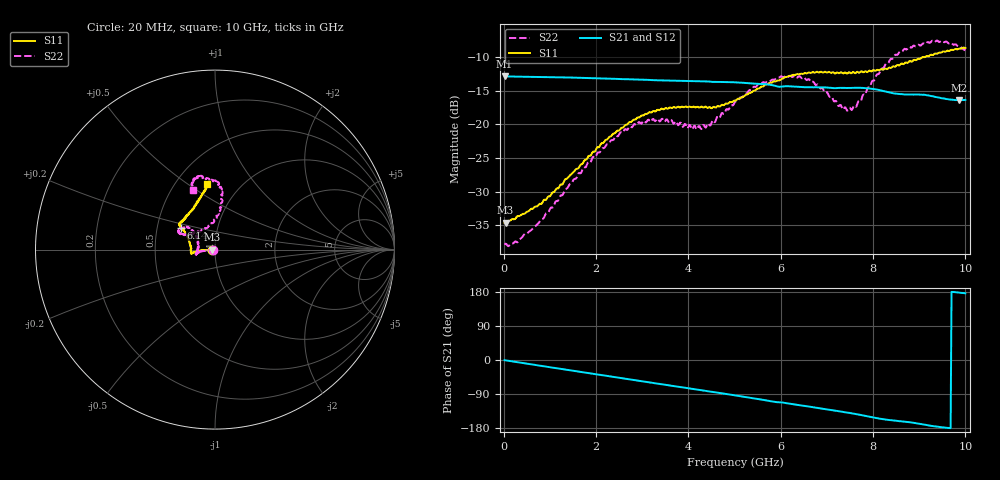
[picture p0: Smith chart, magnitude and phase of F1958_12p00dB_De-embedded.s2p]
! Integrated Device Technology
! Corporate Headquarters
! 6024 Silver Creek Valley Road
! San Jose, CA 95138  USA
! Phone:  1-408-284-8200
! Toll Free:  1-800-223-1366
! Webpage:  http://www.idt.com/
! Timing and RF Division
! 515 Groton Road, Suite 102
! Westford, MA 01886-6024
! Device:  F1958
! Description: 7-bit 0.25 dB Digital Step Attenuator
! Frequency:  0.001 -  6.000 GHz
! Package:  4x4 mm Thin QFN Plastic Package: 24 pin
! Ports:  2 RF, 12 DC
!  Pin  1  = D0
!  Pin  2  = VDD
!  Pin  3  = VMODE
!  Pin  4  = GND
!  Pin  5  = RF1  =  Port 1
!  Pin  6  = GND
!  Pin  7  = GND
!  Pin  8  = GND
!  Pin  9  = GND
!  Pin 10  = GND
!  Pin 11  = GND
!  Pin 12  = GND
!  Pin 13  = GND
!  Pin 14  = RF2  =  Port 2
!  Pin 15  = GND
!  Pin 16  = LE
!  Pin 17  = CLK
!  Pin 18  = DATA
!  Pin 19  = D6
!  Pin 20  = D5
!  Pin 21  = D4
!  Pin 22  = D3
!  Pin 23  = D2
!  Pin 24  = D1
! State:  48
! Atten State:  12.00 dB
! Voltage:  +3.30 Volts
! Current:  0.258 mA
! Data:  The device was measured on a F1958 evaluation board which has
!  individual transmission lines to the RF pins.  Data was collected
!  using a calibrated network analyzer.  The evaluation board was
!  de-embedded using Automatic Fixture Removal (AFR).
!  The reference plane is the edge of the package pin.
! Misc:
!  Action Tracker AT0419
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# GHz S dB R 50
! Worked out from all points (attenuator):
!   500 points, 20 MHz to 10 GHz, reference 50 ohm
!   highest |S21| = -12.84 dB at 20 MHz (marker M1); lowest = -16.4 dB at 9.86 GHz (marker M2)
!   lowest |S11| = -34.6 dB at 40 MHz (marker M3), VSWR 1.04, Z = 48.2 - j0.097 ohm
!   |S11| at or under -10 dB: start of sweep to 9.065 GHz; 9.097628 GHz to 9.109074 GHz (11.45 MHz wide, 0.126 % of centre)
!   |S22| runs from -38.1 to -7.5 dB; largest |S21 - S12| = 0.00067
!   S11 on the Smith chart (normalised r, x): 20 MHz: 0.96, -0.00; 6.14 GHz: 0.66, +0.17; 10 GHz: 0.70, +0.60
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0.02  -34.58 -177.2  -12.84 -0.5  -12.84 -0.5  -37.87 -176.3
0.04  -34.61 -176.9  -12.85 -0.9  -12.84 -0.9  -37.72 -174.5
0.32  -33.61 179.7  -12.89 -6.2  -12.89 -6.2  -37.33 -178.5
0.72  -32.18 -178.1  -12.93 -13.8  -12.92 -13.8  -34.87 -174.6
1.7  -25.87 -176.6  -13.07 -32.1  -13.07 -32.1  -26.79 -174.6
2.6  -20.35 -174.5  -13.26 -48.9  -13.24 -48.9  -20.99 -171.7
2.92  -18.94 -172.4  -13.33 -54.8  -13.31 -54.9  -19.67 -169.0
3.36  -17.86 -170.8  -13.44 -63.0  -13.44 -63.1  -19.40 -165.3
4.3  -17.38 -177.7  -13.58 -80.1  -13.59 -80.2  -20.42 166.0
4.52  -17.52 176.3  -13.67 -84.3  -13.68 -84.4  -19.41 156.6
5.02  -16.45 162.2  -13.74 -93.6  -13.75 -93.6  -16.56 141.0
5.52  -14.65 152.0  -13.96 -103.2  -13.97 -103.2  -13.99 141.0
6.14  -12.91 147.2  -14.31 -114.3  -14.33 -114.3  -12.92 150.8
6.68  -12.25 144.0  -14.47 -124.1  -14.48 -124.1  -13.68 154.4
7.3  -12.23 137.6  -14.56 -136.0  -14.57 -135.8  -17.11 133.1
7.5  -12.28 134.9  -14.58 -139.9  -14.58 -139.8  -17.51 114.6
7.68  -12.25 131.8  -14.54 -143.8  -14.54 -143.8  -16.56 97.5
8.34  -11.57 116.2  -15.23 -158.4  -15.23 -158.5  -10.77 81.7
8.68  -10.91 109.2  -15.54 -162.7  -15.53 -162.8  -8.75 86.3
9.26  -9.63 101.1  -15.78 -173.7  -15.78 -173.8  -7.68 99.5
9.86  -8.73 96.8  -16.40 177.9  -16.43 178.0  -8.44 109.2
10  -8.62 96.9  -16.35 175.9  -16.37 175.9  -8.98 110.2
